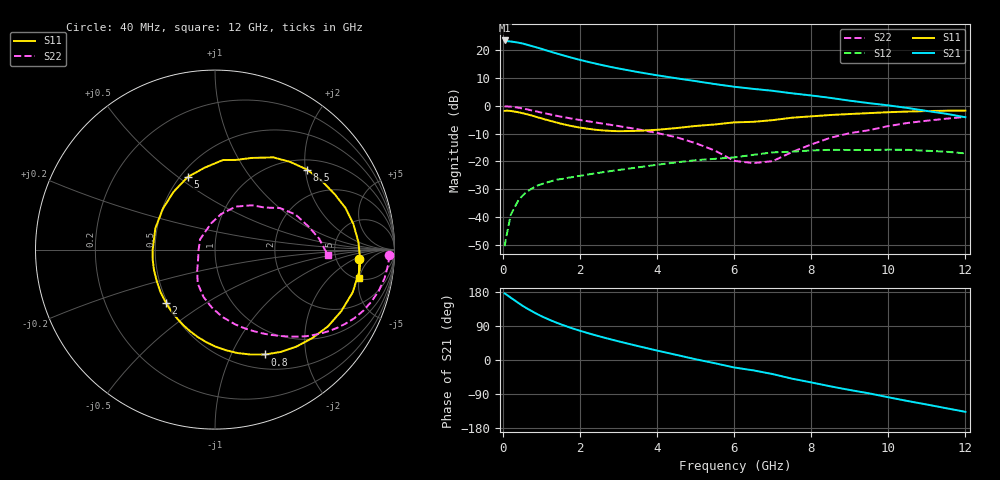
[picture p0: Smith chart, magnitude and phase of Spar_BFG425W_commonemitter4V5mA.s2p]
! Filename: 45bfg425.001
! BFG425W Field C1
! V1=8.213E-001V,V2=4.000E+000V, I1=5.090E-005A, I2=5.010E-003A
# GHz  S  MA  R 50
!  S11  S21  S12  S22
!Freq(GHz)  Mag  Ang  Mag  Ang  Mag  Ang  Mag  Ang
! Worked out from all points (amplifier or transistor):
!   44 points, 40 MHz to 12 GHz, reference 50 ohm
!   highest |S21| = 23.4 dB at 40 MHz (marker M1)
!   |S21| within 3 dB of that: start of sweep to 991.9 MHz
!   unconditionally stable (mu >= 1): 2.468 GHz to end of sweep
!   at 700 MHz: K = 0.36, MSG = 25.9 dB, |S12| = -30.2 dB
!   at 2.4 GHz: K = 0.98, MSG = 19.7 dB, |S12| = -24.3 dB
!   at 12 GHz: K = 1.51, MAG = 2.3 dB, |S12| = -17.1 dB
!   S11 on the Smith chart (normalised r, x): 40 MHz: 8.50, -2.61; 800 MHz: 0.67, -1.36; 2 GHz: 0.49, -0.35; 5 GHz: 0.55, +0.54; 8.5 GHz: 1.24, +2.05; 12 GHz: 5.09, -4.91
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0.04  0.806 -3.8  14.82 175.8  0.003 47.2  0.971 -1.8
0.2  0.803 -17.3  14.19 164.4  0.011 73.5  0.958 -9.6
0.3  0.783 -25.9  13.89 157.4  0.015 70.8  0.941 -14.1
0.5  0.733 -42.2  13.1 143.5  0.024 63.4  0.893 -22.5
0.6  0.706 -49.9  12.54 137.3  0.028 60.0  0.865 -26.2
0.8  0.648 -64.4  11.48 125.8  0.034 53.7  0.806 -32.9
1  0.59 -77.7  10.45 115.5  0.039 48.6  0.751 -38.5
1.3  0.517 -95.6  9.032 102.1  0.045 42.8  0.678 -45.6
1.6  0.458 -112.3  7.869 90.5  0.049 38.6  0.617 -51.5
2  0.404 -132.5  6.628 77.1  0.055 34.6  0.553 -58.5
2.2  0.385 -142.3  6.128 71.0  0.058 32.9  0.525 -61.8
2.6  0.359 -161.1  5.298 59.7  0.064 29.9  0.475 -68.5
3  0.348 -178.9  4.648 49.2  0.07 26.9  0.43 -75.1
3.5  0.353 160.4  4.012 36.8  0.078 22.8  0.377 -83.8
4.5  0.396 125.7  3.103 13.5  0.096 12.5  0.271 -103.7
5  0.432 110.7  2.758 1.9  0.105 5.5  0.212 -117.0
6  0.501 84.9  2.185 -19.7  0.118 -8.1  0.102 -156.1
6.5  0.513 76.9  2.001 -27.4  0.131 -9.2  0.093 -173.6
7.5  0.608 57.7  1.666 -49.3  0.149 -28.2  0.147 98.8
8.5  0.68 40.9  1.379 -69.6  0.161 -45.1  0.266 64.2
10.5  0.784 10.5  0.909 -108.2  0.161 -80.6  0.489 23.6
12  0.817 -11.3  0.62 -136.7  0.139 -111.9  0.629 -2.8
